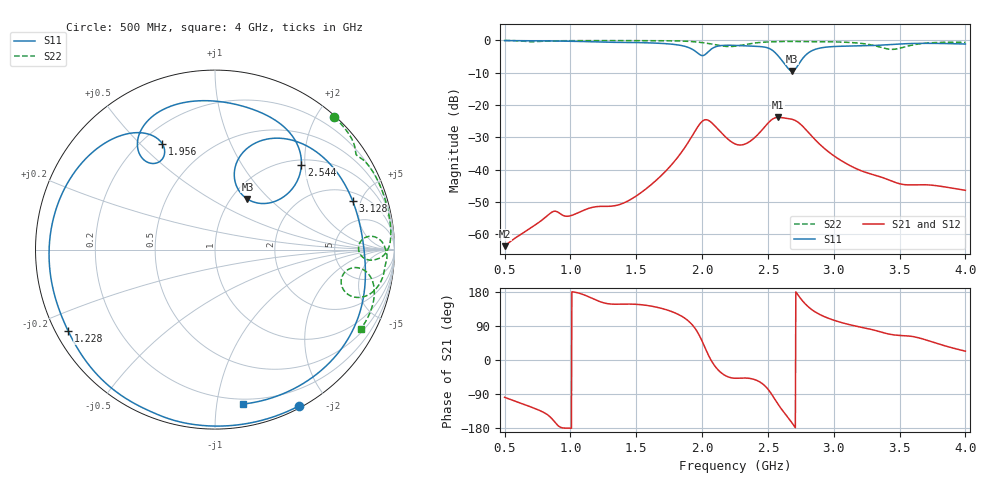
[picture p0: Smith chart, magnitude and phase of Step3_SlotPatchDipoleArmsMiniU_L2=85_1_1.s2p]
! TOUCHSTONE file generated by CST MICROWAVE STUDIO
! Date and time: Tue May 19 02:44:41 2020
! Project name: DualBand_DualMode_Antenna_FD_SteppedDesign.cst
! Parameters = {FPL=20; FPW=20; L=50; ST=10; SW=30; W=52; WF=7; ext=10; gap=1; inset=13}
! Header version: 2015
! Port assignment regex: !\s*Touchstone port\s*([0-9]+)\s*=\s*CST MWS port\s*([0-9]+)\s*\(\"(.*)\"\)(\s*mode\s*([0-9]+))?.*
! Touchstone port assignment:
! Touchstone port 1 = CST MWS port 1 ("")
! Touchstone port 2 = CST MWS port 2 ("")
# GHz S MA R 50
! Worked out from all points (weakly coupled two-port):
!   1006 points, 500 MHz to 4 GHz, reference 50 ohm
!   highest |S21| = -23.83 dB at 2.579 GHz (marker M1); lowest = -63.6 dB at 500 MHz (marker M2)
!   lowest |S11| = -9.5 dB at 2.684 GHz (marker M3), VSWR 2.01, Z = 59.2 + j37.5 ohm
!   |S11| at or under -10 dB: nowhere
!   |S22| runs from -2.8 to -0.1 dB; largest |S21 - S12| = 1.7e-05
!   S11 on the Smith chart (normalised r, x): 500 MHz: 0.02, -1.67; 1.228 GHz: 0.04, -0.26; 1.956 GHz: 0.28, +0.58; 2.544 GHz: 1.11, +1.92; 3.128 GHz: 2.64, +4.24; 4 GHz: 0.16, -1.18
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0.5  0.9886 -61.8  0.000658 -98.5  0.0006579 -98.5  0.9931 48.0
0.787  0.9814 -97.3  0.001684 -136.6  0.001684 -136.6  0.9665 30.9
0.8745  0.9739 -108.3  0.002274 -161.1  0.002274 -161.1  0.9792 27.1
1.0845  0.9565 -134.0  0.002283 174.3  0.002283 174.3  0.9872 19.7
1.228  0.9353 -151.1  0.00271 153.5  0.00271 153.5  0.9881 15.7
1.424  0.9266 -174.3  0.003188 147.6  0.003189 147.6  0.9879 11.1
1.669  0.8996 154.6  0.007393 138.2  0.007394 138.2  0.9845 5.7
1.8475  0.8255 129.8  0.01906 115.0  0.01906 115.0  0.9717 1.4
1.956  0.6595 116.5  0.0424 78.7  0.0424 78.7  0.9425 -1.8
2.019  0.5934 126.0  0.05881 35.1  0.05881 35.1  0.9092 -3.2
2.082  0.7588 124.2  0.05104 -8.4  0.05104 -8.4  0.8684 -3.9
2.25  0.8334 95.6  0.02502 -48.1  0.02502 -48.1  0.8094 2.9
2.446  0.7973 66.2  0.03908 -59.6  0.03909 -59.6  0.9272 3.0
2.544  0.6745 44.5  0.06195 -98.7  0.06195 -98.7  0.9489 0.3
2.579  0.5704 38.9  0.06438 -117.7  0.06437 -117.7  0.9537 -0.5
2.684  0.3346 57.3  0.06003 -166.6  0.06002 -166.6  0.9584 -3.3
2.7505  0.4794 76.2  0.04983 161.4  0.04982 161.4  0.9539 -4.7
2.8345  0.6899 63.7  0.03273 132.6  0.03273 132.6  0.9511 -6.3
3.1285  0.8135 19.5  0.01143 92.5  0.01143 92.5  0.9234 -13.6
3.419  0.8554 -12.0  0.006937 68.4  0.006938 68.4  0.7288 -15.1
3.5835  0.8901 -31.2  0.005816 62.8  0.005815 62.8  0.8322 -7.7
4  0.8747 -79.8  0.004803 23.4  0.004803 23.3  0.9249 -28.5
